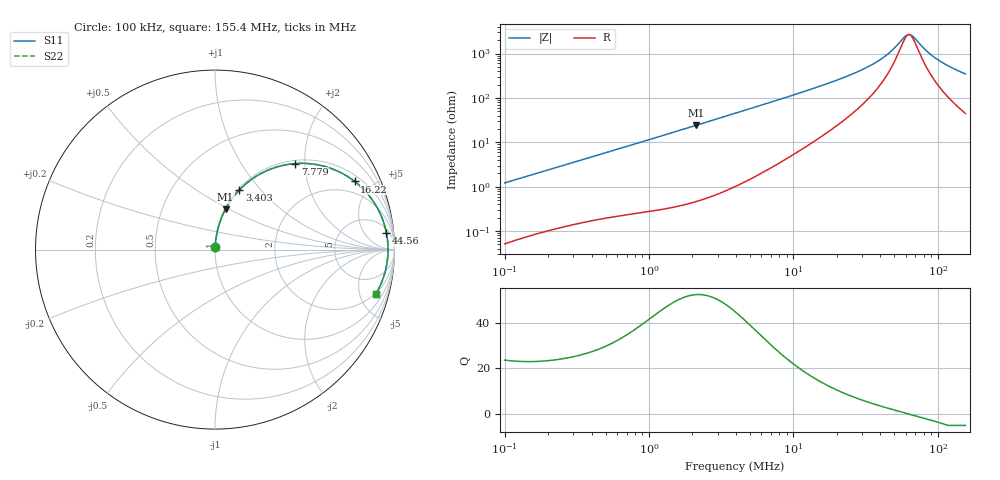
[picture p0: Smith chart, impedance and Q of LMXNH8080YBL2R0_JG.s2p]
! LMXNH8080YBL2R0_JG  S-PARAMETER MODEL  ( General Type )
! Model Generated by TAIYO YUDEN Corporation (http://www.ty-top.com)
! Version 1.0
! TAIYO YUDEN Control No. 191025NI43SB-FBB
! Copyright(c) 2019 TAIYO YUDEN CO.,LTD. All Rights Reserved.
! Product Description (link to TY-COMPAS)
! https://ds.yuden.co.jp/TYCOMPAS/or/detail?pn=LMXNH8080YBL2R0NJG&u=M
! Products Name : Inductors
! Characteristics :
!  Inductance : 2.0 uH , SRF(min) : 50 MHz , DC Resistance(max) : 0.0117 Ohm
!  Rated Current : Saturation :8100 mA , Temp Rise : 6300 mA
!  Case Size : 8.0 x 8.0 / 0.315 x 0.315 [mm/inch] , Thickness : 4.2 / 0.165 [mm/inch]
!  (Conditions: Temperature = 25 degC , DC Bias Current/Voltage = 0A / 0V)
! External Node Assignments :
!  1  o---GGG---o  2
! GND o---------o GND
! Frequency Range : 0.1MHz  -  155.401204MHz  [ 402 STEP ]
# MHz S RI R 50
! Freq[MHz].  S11 Real  S11 Imag  S21 Real  S21 Imag  S12 Real  S12 Imag  S22 Real  S22 Imag
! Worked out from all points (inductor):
!   401 points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, 100 kHz to 155.4 MHz, reference 50 ohm
!   read as one part in series: L = 1.92 uH near 103.7 kHz
!   highest Q = 52.4 at 2.111 MHz (marker M1), where L = 1.82 uH
!   self-resonance near 63.22 MHz
!   S11 on the Smith chart (normalised r, x): 100 kHz: 1.00, +0.02; 3.403 MHz: 1.02, +0.78; 7.779 MHz: 1.06, +1.80; 16.22 MHz: 1.29, +3.93; 44.56 MHz: 8, +18; 155.4 MHz: 1.90, -6.90
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0.1  0.00066 0.0121  0.9993 -0.0121  0.9993 -0.0121  0.00066 0.0121
0.342427  0.00313 0.0398  0.9969 -0.0398  0.9969 -0.0398  0.00313 0.0398
1.172566  0.0205 0.1309  0.9795 -0.1309  0.9795 -0.1309  0.0205 0.1309
2.110832  0.0586 0.2256  0.9414 -0.2256  0.9414 -0.2256  0.0586 0.2256
3.403283  0.1363 0.3328  0.8637 -0.3328  0.8637 -0.3328  0.1363 0.3328
3.942096  0.1741 0.3682  0.8259 -0.3682  0.8259 -0.3682  0.1741 0.3682
5.387211  0.2813 0.4363  0.7187 -0.4363  0.7187 -0.4363  0.2813 0.4363
7.779232  0.4485 0.4796  0.5515 -0.4796  0.5515 -0.4796  0.4485 0.4796
13.49882  0.7093 0.4245  0.2907 -0.4245  0.2907 -0.4245  0.7093 0.4245
16.22117  0.7785 0.3796  0.2215 -0.3796  0.2215 -0.3796  0.7785 0.3796
29.74248  0.9189 0.2038  0.0811 -0.2038  0.0811 -0.2038  0.9189 0.2038
37.07838  0.943 0.1413  0.057 -0.1413  0.057 -0.1413  0.943 0.1413
44.5561  0.9554 0.0914  0.0446 -0.0914  0.0446 -0.0914  0.9554 0.0914
46.22367  0.9572 0.0816  0.0428 -0.0816  0.0428 -0.0816  0.9572 0.0816
58.69305  0.9639 0.0192  0.0361 -0.0192  0.0361 -0.0192  0.9639 0.0192
62.01869  0.9642 0.00494  0.0358 -0.00494  0.0358 -0.00494  0.9642 0.00494
64.33982  0.9642 -0.00456  0.0358 0.00456  0.0358 0.00456  0.9642 -0.00456
67.98542  0.9639 -0.0188  0.0361 0.0188  0.0361 0.0188  0.9639 -0.0188
81.69625  0.9596 -0.0667  0.0404 0.0667  0.0404 0.0667  0.9596 -0.0667
96.38509  0.9514 -0.1108  0.0486 0.1108  0.0486 0.1108  0.9514 -0.1108
120.1582  0.9326 -0.1719  0.0674 0.1719  0.0674 0.1719  0.9326 -0.1719
155.4012  0.8965 -0.2465  0.1035 0.2465  0.1035 0.2465  0.8965 -0.2465
